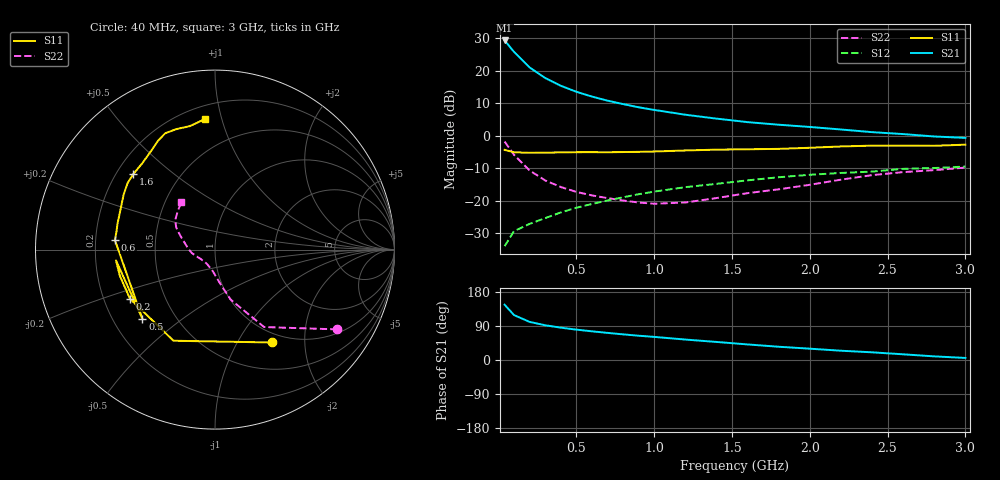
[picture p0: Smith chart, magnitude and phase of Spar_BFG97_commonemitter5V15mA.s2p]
! Filename:  BFG97A.S2P  Version:  2.0
! NXP part #: BFG97  Date: Jul 1990
! Bias condition: Vce=5V, Ic=15mA
#  MHz  S  MA  R  50
! Freq  S11  S21  S12  S22  !GUM [dB]
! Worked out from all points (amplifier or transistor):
!   21 points, 40 MHz to 3 GHz, reference 50 ohm
!   highest |S21| = 29.3 dB at 40 MHz (marker M1)
!   |S21| within 3 dB of that: start of sweep to 91.64 MHz
!   unconditionally stable (mu >= 1): 432 MHz to end of sweep
!   at 300 MHz: K = 0.91, MSG = 21.6 dB, |S12| = -25.4 dB
!   at 1 GHz: K = 1.14, MAG = 10.3 dB, |S12| = -17.2 dB
!   at 3 GHz: K = 1.06, MAG = 2.9 dB, |S12| = -9.5 dB
!   S11 on the Smith chart (normalised r, x): 40 MHz: 0.86, -1.41; 200 MHz: 0.31, -0.24; 500 MHz: 0.32, -0.36; 600 MHz: 0.28, +0.04; 1.6 GHz: 0.27, +0.37; 3 GHz: 0.28, +0.89
40  0.607 -58.5  29.33 145.9  0.02 66.5  0.814 -33.1
100  0.558 -114.5  19.63 118.7  0.034 51.8  0.511 -57.6
200  0.547 -150.0  11.3 100.6  0.044 51.3  0.293 -72.5
300  0.55 -164.7  7.769 91.7  0.054 54.5  0.206 -79.7
400  0.555 -173.8  5.902 85.4  0.066 57.2  0.163 -85.5
500  0.559 -136.3  4.765 80.2  0.078 59.2  0.137 -91.1
600  0.56 174.6  4.021 75.7  0.089 60.5  0.121 -95.8
700  0.558 169.7  3.478 71.6  0.101 61.6  0.11 -101.7
800  0.562 165.2  3.079 67.7  0.113 61.7  0.101 -108.1
900  0.566 160.6  2.75 64.1  0.126 61.3  0.094 -115.4
1000  0.573 156.5  2.503 61.0  0.138 61.4  0.09 -124.9
1200  0.594 149.0  2.111 54.0  0.162 59.7  0.094 -144.7
1400  0.612 142.7  1.838 47.7  0.182 57.8  0.11 -160.4
1600  0.62 137.2  1.624 41.1  0.206 56.6  0.131 -171.8
1800  0.629 130.1  1.481 35.0  0.23 52.9  0.15 177.5
2000  0.654 123.1  1.368 29.9  0.251 51.7  0.176 166.5
2200  0.685 117.5  1.25 24.5  0.268 49.0  0.211 157.5
2400  0.705 113.2  1.138 20.3  0.281 47.9  0.248 150.5
2600  0.705 107.9  1.063 15.0  0.31 44.3  0.276 143.5
2800  0.702 101.5  0.976 9.6  0.319 39.5  0.296 134.9
3000  0.73 94.3  0.928 5.4  0.336 38.0  0.324 125.6
